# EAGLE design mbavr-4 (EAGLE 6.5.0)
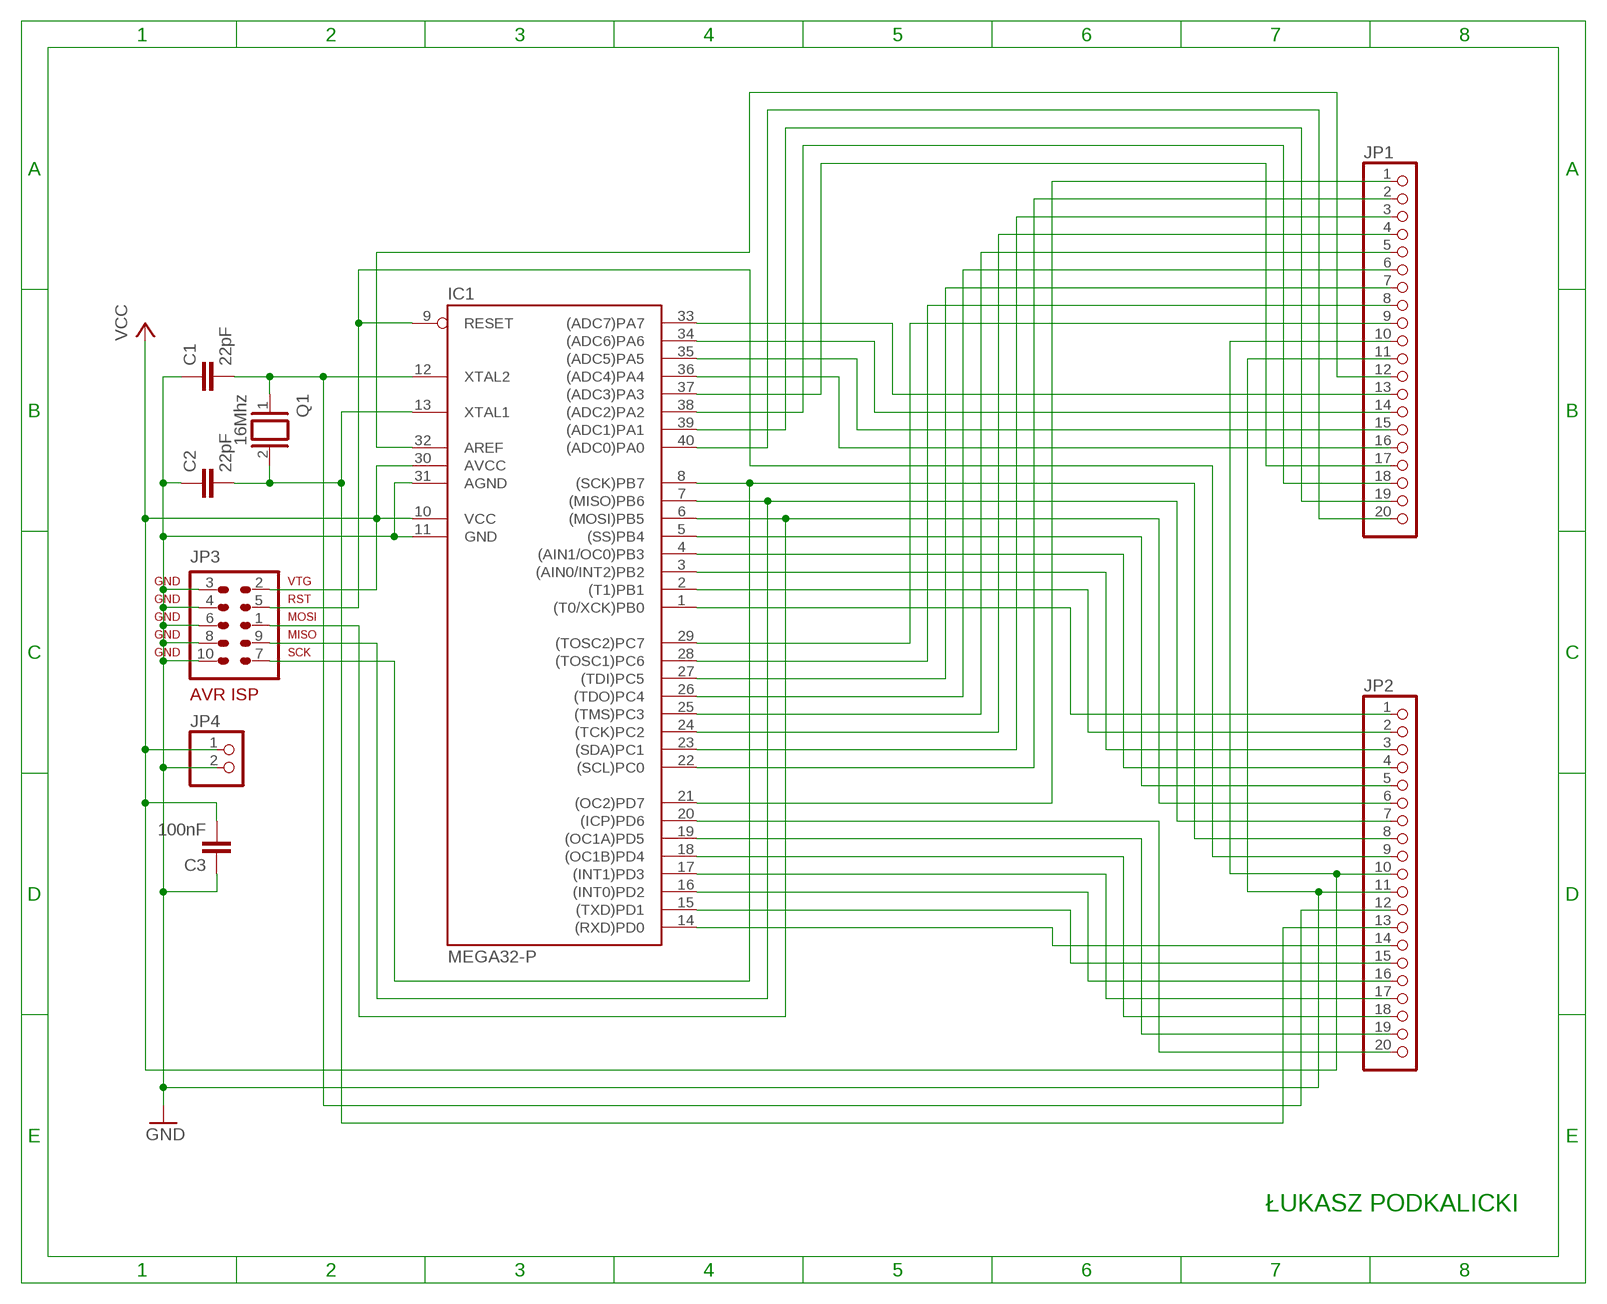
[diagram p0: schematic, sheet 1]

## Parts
C1  22pF  C-EU050-025X075  [C050-025X075]
C2  22pF  C-EU050-025X075  [C050-025X075]
C3  100nF  C-EU050-025X075  [C050-025X075]
IC1  MEGA32-P  [DIL40]
JP1  PINHD-1X20  [1X20]
JP2  PINHD-1X20  [1X20]
JP3  AVR-ISP-10  [AVR-ISP-10]
JP4  PINHD-1X2  [1X02]
Q1  16Mhz  XTAL/S  [QS]

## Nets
GND: C1.1 C2.1 C3.1 IC1.11(GND) IC1.31(AGND) JP1.11 JP2.11 JP3.3 JP3.4 JP3.6 JP3.8 JP3.10 JP4.2
N$1: C2.2 IC1.13(XTAL1) JP2.13 Q1.2
N$2: C1.2 IC1.12(XTAL2) JP2.12 Q1.1
N$5: IC1.1((T0/XCK)PB0) JP2.1
N$6: IC1.2((T1)PB1) JP2.2
N$7: IC1.3((AIN0/INT2)PB2) JP2.3
N$8: IC1.4((AIN1/OC0)PB3) JP2.4
N$9: IC1.5((SS)PB4) JP2.5
N$10: IC1.6((MOSI)PB5) JP2.6 JP3.1
N$11: IC1.7((MISO)PB6) JP2.7 JP3.9
N$12: IC1.8((SCK)PB7) JP2.8 JP3.7
N$14: IC1.14((RXD)PD0) JP2.14
N$15: IC1.15((TXD)PD1) JP2.15
N$16: IC1.16((INT0)PD2) JP2.16
N$17: IC1.17((INT1)PD3) JP2.17
N$18: IC1.18((OC1B)PD4) JP2.18
N$19: IC1.19((OC1A)PD5) JP2.19
N$20: IC1.20((ICP)PD6) JP2.20
N$21: IC1.21((OC2)PD7) JP1.1
N$22: IC1.22((SCL)PC0) JP1.2
N$23: IC1.23((SDA)PC1) JP1.3
N$24: IC1.24((TCK)PC2) JP1.4
N$25: IC1.25((TMS)PC3) JP1.5
N$26: IC1.26((TDO)PC4) JP1.6
N$27: IC1.27((TDI)PC5) JP1.7
N$28: IC1.28((TOSC1)PC6) JP1.8
N$29: IC1.29((TOSC2)PC7) JP1.9
N$30: IC1.33((ADC7)PA7) JP1.13
N$31: IC1.34((ADC6)PA6) JP1.14
N$32: IC1.35((ADC5)PA5) JP1.15
N$33: IC1.36((ADC4)PA4) JP1.16
N$34: IC1.37((ADC3)PA3) JP1.17
N$35: IC1.38((ADC2)PA2) JP1.18
N$36: IC1.39((ADC1)PA1) JP1.19
N$37: IC1.40((ADC0)PA0) JP1.20
N$38: IC1.32(AREF) JP1.12
N$39: IC1.9(RESET) JP2.9 JP3.5
VCC: C3.2 IC1.10(VCC) IC1.30(AVCC) JP1.10 JP2.10 JP3.2 JP4.1

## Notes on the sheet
- ŁUKASZ PODKALICKI

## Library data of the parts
C1-C3 = rcl:C-EU: CAPACITOR, European symbol
IC1 = avr-7:MEGA32-P: MICROCONTROLLER 32 Kbytes FLASH 2 Kbytes SRAM 1 Kbytes EEPROM USART 8-channel 10 bit ADC
JP1 JP2 = pinhead:PINHD-1X20: PIN HEADER
JP3 = avr-7:AVR-ISP-10: AVR ISP-10 Serial Programming Header
JP4 = pinhead:PINHD-1X2: PIN HEADER
Q1 = special:XTAL/S: CRYSTAL

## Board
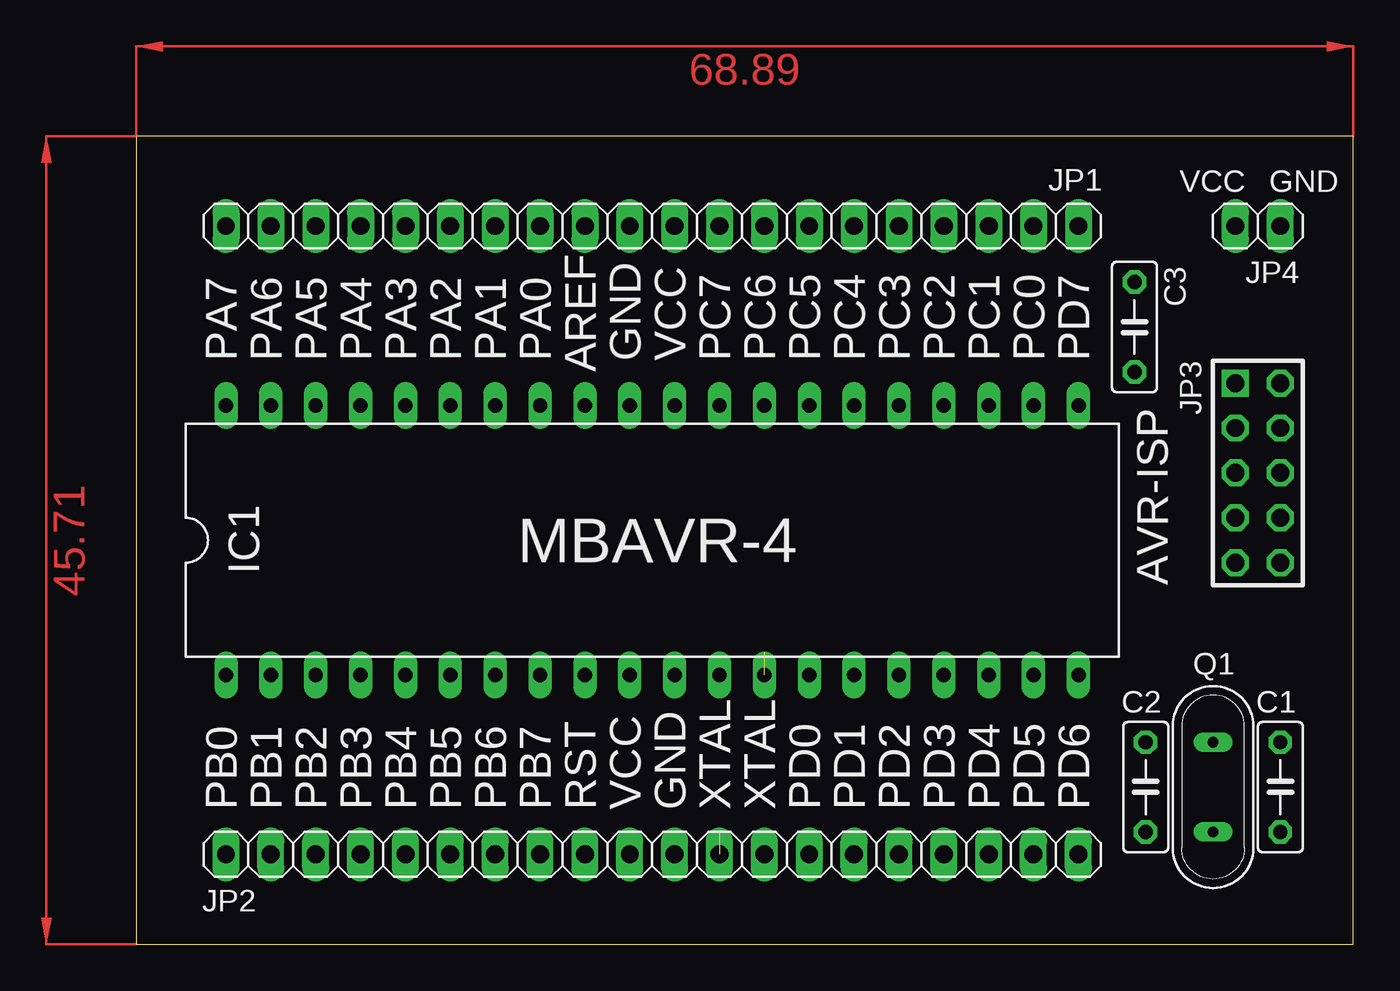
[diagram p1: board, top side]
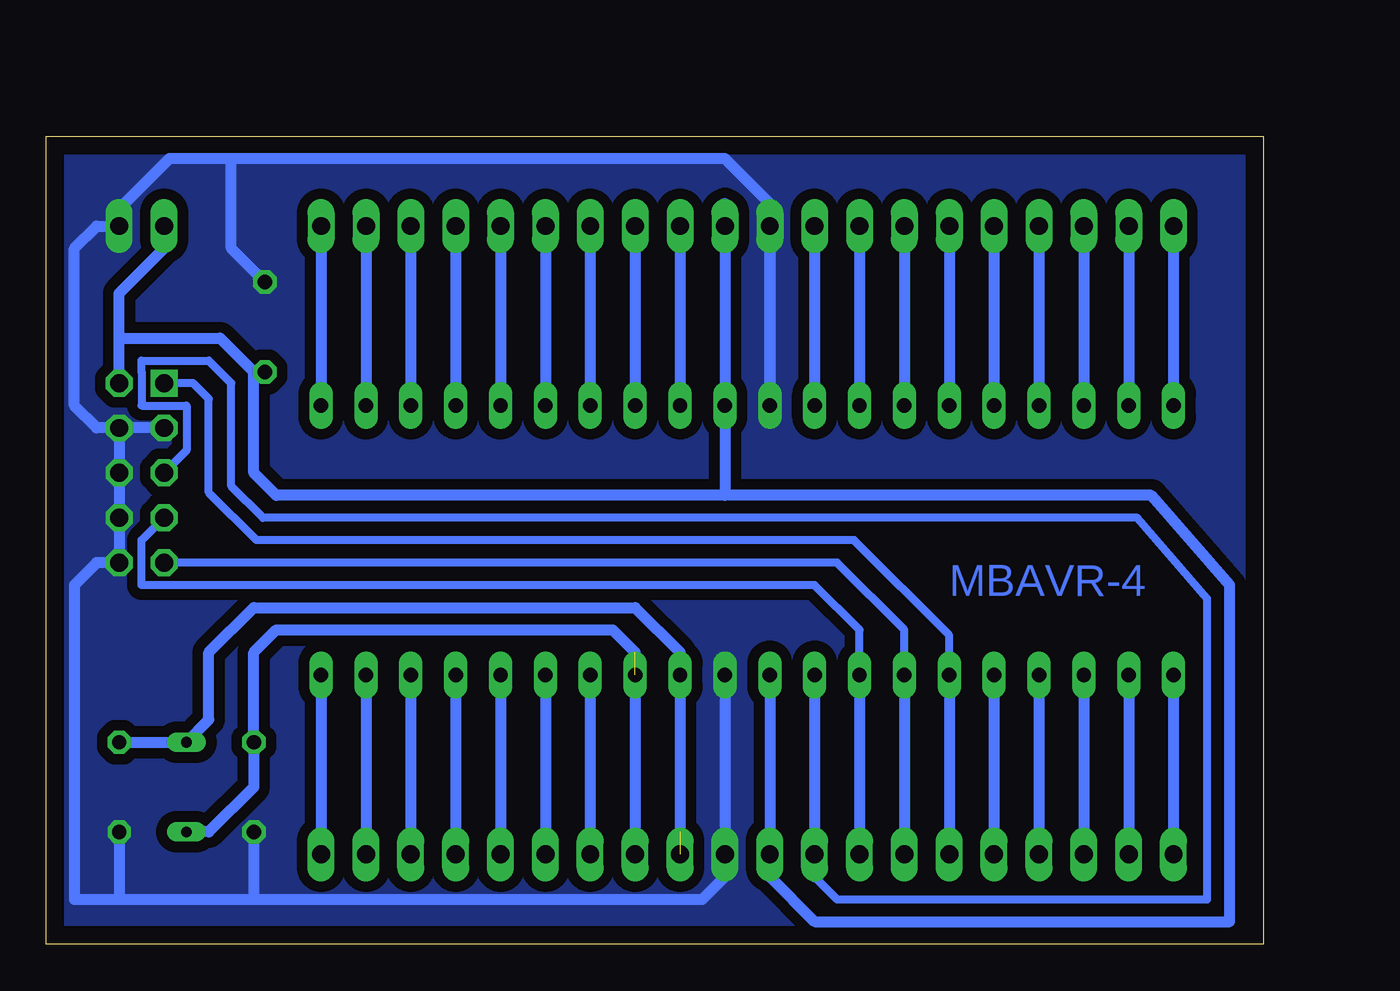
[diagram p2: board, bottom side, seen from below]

Size 68.89 x 45.71 mm. Coordinates in mm from the lower left corner, seen from the top.
Outline: 0,0 68.89,0 68.89,45.71 0,45.71 0,0
Copper layers (1*16): Top 0.035mm / dielectric 1.5mm / Bottom 0.035mm
Design rules "default": minimum track width 10mil, minimum drill 24mil, track to track 8mil, track to pad 8mil, pad to pad 8mil, via to via 8mil, smd to smd 8mil, copper to edge 40mil, drill to drill 8mil, minimum pad ring 10mil, minimum via ring 8mil, stop-mask expansion 4mil, vias tented up to drill 0mil, thermal gap 10mil

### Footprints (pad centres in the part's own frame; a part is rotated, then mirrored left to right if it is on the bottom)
C050-025X075 = drill 0.813 octagon: 1 -2.54,0; 2 2.54,0
DIL40 = drill 0.813 long: 1 -24.13,-7.62; 2 -21.59,-7.62; 3 -19.05,-7.62; 4 -16.51,-7.62; 5 -13.97,-7.62; 6 -11.43,-7.62; 7 -8.89,-7.62; 8 -6.35,-7.62; 9 -3.81,-7.62; 10 -1.27,-7.62; 11 1.27,-7.62; 12 3.81,-7.62; 13 6.35,-7.62; 14 8.89,-7.62; 15 11.43,-7.62; 16 13.97,-7.62; 17 16.51,-7.62; 18 19.05,-7.62; 19 21.59,-7.62; 20 24.13,-7.62; 21 24.13,7.62; 22 21.59,7.62; 23 19.05,7.62; 24 16.51,7.62; 25 13.97,7.62; 26 11.43,7.62; 27 8.89,7.62; 28 6.35,7.62; 29 3.81,7.62; 30 1.27,7.62; 31 -1.27,7.62; 32 -3.81,7.62; 33 -6.35,7.62; 34 -8.89,7.62; 35 -11.43,7.62; 36 -13.97,7.62; 37 -16.51,7.62; 38 -19.05,7.62; 39 -21.59,7.62; 40 -24.13,7.62
1X20 = drill 1.016 long: 1 -24.13,0; 2 -21.59,0; 3 -19.05,0; 4 -16.51,0; 5 -13.97,0; 6 -11.43,0; 7 -8.89,0; 8 -6.35,0; 9 -3.81,0; 10 -1.27,0; 11 1.27,0; 12 3.81,0; 13 6.35,0; 14 8.89,0; 15 11.43,0; 16 13.97,0; 17 16.51,0; 18 19.05,0; 19 21.59,0; 20 24.13,0
AVR-ISP-10 = drill 1.016 square: 1 -5.08,-1.27 | drill 1.016 octagon: 2 -5.08,1.27; 3 -2.54,-1.27; 4 -2.54,1.27; 5 0,-1.27; 6 0,1.27; 7 2.54,-1.27; 8 2.54,1.27; 9 5.08,-1.27; 10 5.08,1.27
1X02 = drill 1.016 long: 1 -1.27,0; 2 1.27,0
QS = drill 0.61 long: 1 -2.54,0; 2 2.54,0

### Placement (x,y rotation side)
C1  64.77,8.89 90 top
C2  57.15,8.89 90 top
C3  56.52,34.92 270 top
IC1  29.21,22.86 0 top
JP1  29.21,40.64 180 top
JP2  29.21,5.08 0 top
JP3  63.5,26.67 270 top
JP4  63.5,40.64 0 top
Q1  60.96,8.89 270 top

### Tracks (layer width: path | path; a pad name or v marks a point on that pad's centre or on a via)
GND
  Bottom 0.61: JP1.11 IC1.31 27.94,41.91 30.48,44.45 58.42,44.45 | IC1.11 JP2.11 30.48,3.81 31.75,2.54 57.15,2.54 | JP3.4 66.04,29.21 67.31,30.48 67.31,39.37 66.04,40.64 JP4.2 64.77,41.61 61.93,44.45 58.42,44.45 | JP3.3 JP3.4 | JP3.4 JP3.6 JP3.8 JP3.10 66.04,21.59 67.31,20.32 67.31,2.54 64.77,2.54 | 64.77,2.54 57.15,2.54 | C2.1 57.15,2.54 | C1.1 64.77,2.54 | C3.1 58.42,39.37 58.42,44.45
  pour Bottom (isolate 0.61, no thermals): -1.27,48.26 72.39,48.26 72.39,-1.27 -1.27,-1.27
N$1  (1 unrouted)
  Bottom 0.61: IC1.13 JP2.13 | 35.56,16.51 36.83,17.78 55.88,17.78 57.15,16.51 C2.2 57.15,8.89 59.69,6.35 Q1.2
N$2  (1 unrouted)
  Bottom 0.61: 33.02,6.35 IC1.12 33.02,16.51 35.56,19.05 57.15,19.05 59.69,16.51 59.69,12.7 Q1.1 C1.2
N$5
  Bottom 0.61: IC1.1 JP2.1
N$6
  Bottom 0.61: IC1.2 JP2.2
N$7
  Bottom 0.61: IC1.3 JP2.3
N$8
  Bottom 0.61: IC1.4 JP2.4
N$9
  Bottom 0.61: IC1.5 JP2.5
N$10
  Bottom 0.457: IC1.6 17.78,17.47 23.17,22.86 57,22.86 59.69,25.55 59.69,30.85 60.59,31.75 JP3.1
  Bottom 0.61: IC1.6 JP2.6
N$11
  Bottom 0.457: IC1.7 20.32,17.78 24.13,21.59 JP3.9
  Bottom 0.61: IC1.7 JP2.7
N$12
  Bottom 0.457: IC1.8 22.86,17.78 25.4,20.32 63.5,20.32 63.5,22.86 JP3.7
  Bottom 0.61: IC1.8 JP2.8
N$14
  Bottom 0.61: IC1.14 JP2.14
N$15
  Bottom 0.61: IC1.15 JP2.15
N$16
  Bottom 0.61: IC1.16 JP2.16
N$17
  Bottom 0.61: IC1.17 JP2.17
N$18
  Bottom 0.61: IC1.18 JP2.18
N$19
  Bottom 0.61: IC1.19 JP2.19
N$20
  Bottom 0.61: IC1.20 JP2.20
N$21
  Bottom 0.61: JP1.1 IC1.21
N$22
  Bottom 0.61: JP1.2 IC1.22
N$23
  Bottom 0.61: JP1.3 IC1.23
N$24
  Bottom 0.61: JP1.4 IC1.24
N$25
  Bottom 0.61: JP1.5 IC1.25
N$26
  Bottom 0.61: JP1.6 IC1.26
N$27
  Bottom 0.61: JP1.7 IC1.27
N$28
  Bottom 0.61: JP1.8 IC1.28
N$29
  Bottom 0.61: JP1.9 IC1.29
N$30
  Bottom 0.61: JP1.13 IC1.33
N$31
  Bottom 0.61: JP1.14 IC1.34
N$32
  Bottom 0.61: JP1.15 IC1.35
N$33
  Bottom 0.61: JP1.16 IC1.36
N$34
  Bottom 0.61: JP1.17 IC1.37
N$35
  Bottom 0.61: JP1.18 IC1.38
N$36
  Bottom 0.61: JP1.19 IC1.39
N$37
  Bottom 0.61: JP1.20 IC1.40
N$38
  Bottom 0.61: JP1.12 IC1.32
N$39
  Bottom 0.457: 25.4,3.81 24.13,2.54 3.17,2.54 3.17,19.55 7.12,24.13 56.62,24.13 58.42,25.93 58.42,31.75 59.69,33.02 63.5,33.02 63.5,32.38 63.5,30.48 60.96,30.48 60.96,27.94 JP3.5
  Bottom 0.61: IC1.9 JP2.9 25.4,3.81
VCC
  Bottom 0.61: JP2.10 IC1.10 27.94,3.81 25.4,1.27 1.91,1.27 1.91,20.32 6.35,25.4 30.48,25.4 | 30.48,41.91 JP1.10 IC1.30 30.48,25.4 | JP3.2 64.77,34.29 | 64.77,34.29 64.77,36.83 62.23,39.37 JP4.1 | C3.2 57.15,32.38 | 57.15,32.38 59.05,34.29 64.77,34.29 | 30.48,25.4 55.88,25.4 57.15,26.67 57.15,32.38
(copper drawn outside any net)
  shapes: Top area x2

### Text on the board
Bottom: MBAVR-4
tNames: VCC | GND | PA7 | PA6 | PA5 | PA4 | PA3 | PA2 | PA1 | PA0 | GND | VCC | PC7 | PC6 | PC5 | PC4 | PC3 | PC2 | PC1 | PC0 | PD7 | AREF | MBAVR-4 | AVR-ISP | PB0 | PB1 | PB2 | PB3 | PB4 | PB5 | PB6 | PB7 | RST | VCC | GND | XTAL | XTAL | PD0 | PD1 | PD2 | PD3 | PD4 | PD5 | PD6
